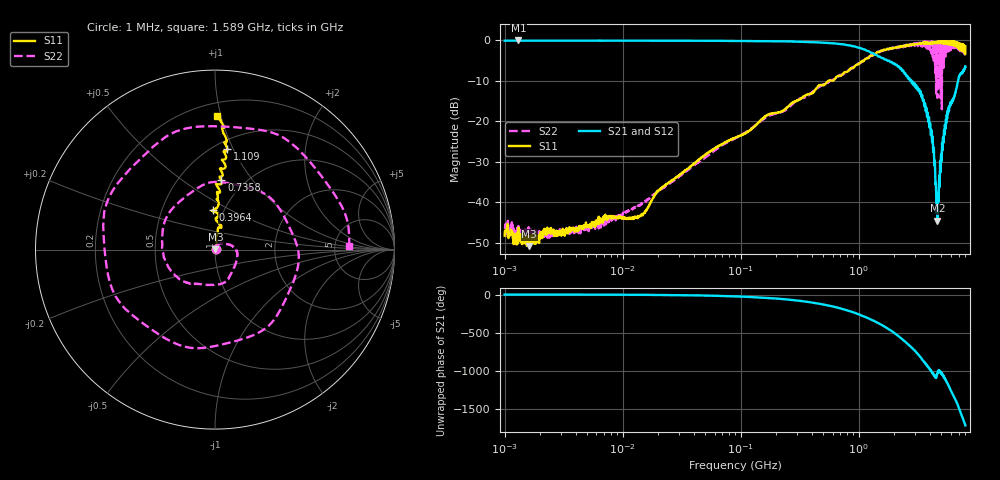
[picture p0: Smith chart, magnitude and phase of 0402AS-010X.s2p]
!s-Parameter Generated by FASTRON Sdn. Bhd.
!FASTRON P/N : 0402AS-010X
!Keysight Technologies: E5071C_MY46733604_B.14.02
!Date: Mon Dec 01 10:30:10 2025
!Version  :Rev00  Mon Dec 01 10:30:10 2025
!Data & Calibration Information:
!Freq  S11:SOLT2(ON)  S21:SOLT2(ON)  S12:SOLT2(ON)  S22:SOLT2(ON)
!PortZ  Port1:50+j0  Port2:50+j0
!When reading reference impedance value at option line is always used.
! Remarks : This data is being provided solely for informational purposes.
# Hz S dB R 50
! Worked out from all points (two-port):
!   1601 points, 1 MHz to 8 GHz, reference 50 ohm
!   highest |S21| = 0.01 dB at 1.31 MHz (marker M1); lowest = -44.6 dB at 4.633 GHz (marker M2)
!   |S21| within 3 dB of the highest: start of sweep to 1.257 GHz
!   lowest |S11| = -50.9 dB at 1.614 MHz (marker M3), VSWR 1.01, Z = 50.3 + j0.132 ohm
!   |S11| at or under -10 dB: start of sweep to 552.2 MHz
!   |S22| runs from -49.3 to 0.0 dB; largest |S21 - S12| = 0.016
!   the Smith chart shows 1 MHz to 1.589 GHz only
!   S11 on the Smith chart (normalised r, x): 1 MHz: 1.01, +0.00; 396.4 MHz: 0.89, +0.41; 735.8 MHz: 0.79, +0.72; 1.109 GHz: 0.58, +0.95; 1.589 GHz: 0.29, +0.97
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1000000  -48.30 16.4  -0.05 -0.3  -0.04 -0.3  -46.20 16.9
1310238  -46.30 13.0  0.01 -0.5  -0.02 -0.4  -45.90 -2.4
1613744  -50.90 27.5  -0.05 -0.4  -0.04 -0.5  -47.30 -7.3
4479405  -46.00 35.6  -0.05 -1.2  -0.04 -1.2  -46.70 42.3
2.00676e7  -37.10 58.3  -0.05 -5.4  -0.05 -5.3  -37.30 67.9
8.994653e7  -24.10 87.1  -0.10 -23.7  -0.10 -23.7  -24.20 31.7
3.963765e8  -13.20 92.8  -0.38 -103.0  -0.38 -103.0  -13.00 -122.0
4.006501e8  -13.10 91.7  -0.39 -104.0  -0.38 -104.0  -12.90 -124.0
7.358266e8  -8.21 84.8  -0.95 169.0  -0.95 169.0  -8.41 73.1
1.108954e9  -4.96 83.0  -2.20 73.2  -2.20 73.1  -4.93 -119.0
1.395953e9  -3.25 85.9  -3.53 2.7  -3.53 2.6  -3.22 96.2
1.589302e9  -2.56 89.2  -4.36 -43.0  -4.37 -43.2  -2.52 1.6
1.7949e9  -2.12 93.0  -4.97 -92.0  -4.98 -92.2  -2.21 -100.0
2.125126e9  -1.60 98.3  -6.32 -174.0  -6.32 -174.0  -1.61 92.8
2.486897e9  -1.27 103.0  -8.19 98.2  -8.17 98.1  -1.56 -90.0
2.853703e9  -1.10 110.0  -10.20 17.2  -10.20 16.9  -1.11 101.0
3.203473e9  -0.79 117.0  -12.50 -66.9  -12.50 -67.3  -0.60 -77.6
3.568312e9  -0.47 128.0  -15.70 -162.0  -15.70 -162.0  -1.14 77.3
3.933151e9  -0.71 130.0  -19.00 119.0  -19.00 118.0  -1.88 -77.6
4.296652e9  -0.62 138.0  -27.00 45.7  -27.00 45.3  -0.28 114.0
4.632554e9  -0.42 140.0  -44.60 44.7  -44.80 44.9  -14.20 157.0
8e9  -1.52 -111.0  -6.57 89.7  -6.59 89.3  -3.28 124.0
